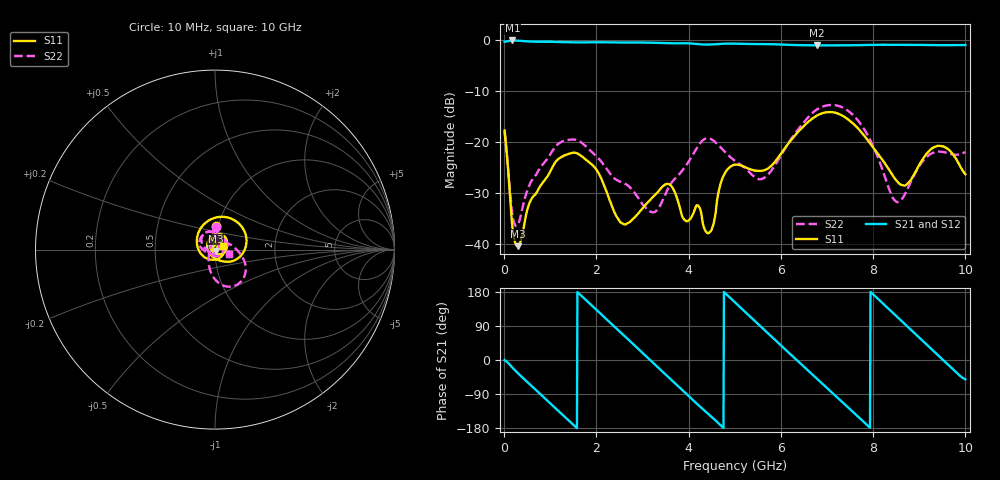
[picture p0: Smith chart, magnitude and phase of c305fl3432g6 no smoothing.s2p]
!Agilent Technologies,N5234A,MY52241123,A.10.00.00
!Agilent N5234A: A.10.00.00
!Date: Wednesday, April 24, 2019 09:08:53
!Correction: S11(Full 2 Port(1,2))
!S21(Full 2 Port(1,2))
!S12(Full 2 Port(1,2))
!S22(Full 2 Port(1,2))
!S2P File: Measurements: S11, S21, S12, S22:
# Hz S  dB  R 50
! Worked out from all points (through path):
!   1001 points, 10 MHz to 10 GHz, reference 50 ohm
!   highest |S21| = -0.11 dB at 179.8 MHz (marker M1); lowest = -1.1 dB at 6.783 GHz (marker M2)
!   group delay of S21, straight-line fit = 315 ps
!   lowest |S11| = -40.4 dB at 289.7 MHz (marker M3), VSWR 1.02, Z = 50.5 - j0.819 ohm
!   |S11| at or under -10 dB: start of sweep to end of sweep
!   |S22| runs from -36.4 to -12.7 dB; largest |S21 - S12| = 0.0019
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1e7  -17.75 88.2  -0.36 -0.2  -0.36 -0.1  -17.89 88.1
1.7983e8  -36.72 22.7  -0.11 -20.4  -0.11 -20.4  -34.26 19.9
2.8972e8  -40.36 -57.7  -0.15 -33.7  -0.14 -33.7  -36.27 -46.6
9.2908e8  -26.85 122.1  -0.37 -106.2  -0.37 -106.2  -23.37 179.0
1.67833e9  -22.73 22.7  -0.49 169.0  -0.49 169.0  -20.10 95.8
2.09791e9  -26.96 -33.6  -0.46 121.3  -0.46 121.3  -23.73 37.4
2.44756e9  -34.71 -111.3  -0.51 81.5  -0.50 81.5  -27.44 -34.5
2.93707e9  -33.62 104.4  -0.50 26.0  -0.50 26.0  -31.27 -138.8
3.34666e9  -29.61 81.0  -0.59 -20.9  -0.59 -20.9  -32.89 -153.9
4.06594e9  -34.61 45.4  -0.71 -102.7  -0.71 -102.7  -22.83 160.4
4.46554e9  -37.57 -122.8  -0.90 -146.6  -0.90 -146.6  -19.33 112.6
5.005e9  -24.41 45.4  -0.73 151.9  -0.73 151.9  -23.67 85.9
5.7043e9  -25.24 -83.9  -0.82 72.3  -0.82 72.3  -26.49 61.1
6.2038e9  -19.80 166.1  -0.98 15.5  -0.98 15.5  -19.64 9.0
6.67333e9  -15.46 99.3  -1.07 -37.1  -1.07 -37.1  -14.38 -27.1
6.78322e9  -14.81 84.9  -1.08 -49.4  -1.08 -49.3  -13.60 -35.0
7.24276e9  -14.44 25.6  -1.07 -100.9  -1.07 -100.9  -12.90 -65.3
7.72228e9  -17.83 -26.2  -1.00 -155.0  -1.00 -155.0  -16.36 -93.9
8.34166e9  -25.33 -81.5  -0.95 134.2  -0.95 134.3  -29.09 -154.7
8.8012e9  -27.60 179.4  -0.96 81.6  -0.96 81.6  -28.07 122.2
9.3007e9  -21.09 80.2  -1.02 24.5  -1.02 24.5  -22.08 86.7
1e10  -26.28 26.9  -1.01 -51.1  -1.01 -51.1  -21.95 -19.2
